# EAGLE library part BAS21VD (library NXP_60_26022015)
High-voltage switching diodes Triple high-voltage switching diodes, encapsulated in a SOT457 (SC-74) small Surface-Mounted Device (SMD) plastic package. AAL Eindhoven MK
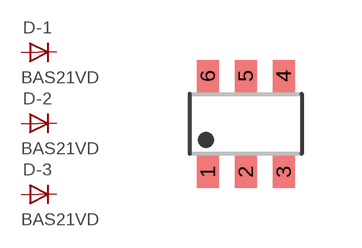
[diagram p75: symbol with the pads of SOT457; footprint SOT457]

Designator prefix D; gates -1=DIODE -2=DIODE -3=DIODE

## BAS21VD  [SOT457]
1  -1:K  pas
2  -2:K  pas
3  -3:K  pas
4  -3:A  pas
5  -2:A  pas
6  -1:A  pas

## Footprint SOT457 (pad centres in mm)
SOT457 TSOP6: Plastic surface-mounted package; 6 lead JEIDA: SC73 A.K.A. SOT23-6
smd 0.55 x 0.8: 1 -0.95,-1.2; 2 0,-1.2; 3 0.95,-1.2; 4 0.95,1.2; 5 0,1.2; 6 -0.95,1.2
